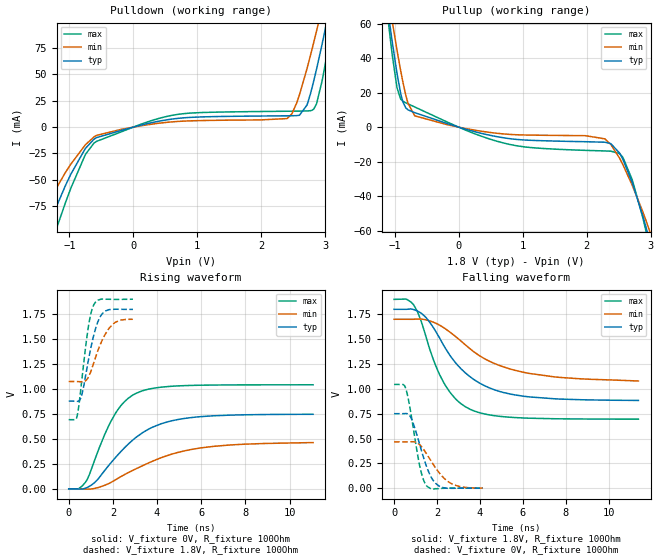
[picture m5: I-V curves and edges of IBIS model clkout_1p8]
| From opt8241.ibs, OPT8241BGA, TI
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|   clkout_1p8 Model
[Model]   clkout_1p8
Model_type   Output
Polarity   Non-Inverting
Vmeas = 0.9
Vref = 0
Cref = 2pF
Rref = 250
|   typ   min   max
|   (nom PVT)   (fast PVT)   (slow PVT)
C_comp   2.233e-12   2.012e-12   2.445e-12
| Where nom  PVT is Nominal Process, 1.8V, 27C
|   Fast PVT is Strong Process,  1.9V, -40C
|   Slow PVT is Weak Process,   1.7V, 125C
[Voltage Range]   1.8   1.7   1.9
|Junction Temperature
[Temperature Range]   27   125   -40
[Pullup Reference]   1.8   1.7   1.9
[Pulldown Reference]   0   0   0
[Power Clamp Reference]   1.8   1.7   1.9
[GND Clamp Reference]   0   0   0
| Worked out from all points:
|   slope of the pulldown table from 0 to 0.27 V, typ, clamps not added: 67 ohm
|   slope of the pullup table from 0 to 0.27 V, typ, clamps not added: 96 ohm
|   falling waveform, V_fixture 1.8V, R_fixture 100Ohm: 20-80 % time 2.09ns typ, 2.79ns min, 1.42ns max; typ from 1.8 V to 0.884 V
|   rising waveform, V_fixture 0V, R_fixture 100Ohm: 20-80 % time 2.11ns typ, 2.92ns min, 1.32ns max; typ from 0 V to 0.747 V
|   rising waveform, V_fixture 1.8V, R_fixture 100Ohm: 20-80 % time 522ps typ, 686ps min, 403ps max; typ from 0.879 V to 1.8 V
|   falling waveform, V_fixture 0V, R_fixture 100Ohm: 20-80 % time 669ps typ, 935ps min, 493ps max; typ from 0.75 V to 0 V
[Pulldown]
|   Voltage   I(typ)   I(min)   I(max)
-1.8V     -252mA     -148.4mA   -354.1mA
-1.551V   -125.9mA   -94.92mA   -164.8mA
-1.06V    -55.32mA   -42.92mA   -71.6mA
-572.4mV  -9.892mA   -7.778mA   -13.42mA
682mV     8.222mA    5.348mA    11.98mA
2.402V    10.74mA    8.113mA    15.09mA
2.596V    11.26mA    30.56mA    15.21mA
2.79V     36.73mA    73.35mA    15.93mA
2.864V    55.26mA    91.37mA    22.36mA
2.968V    83.99mA    117.5mA    49.6mA
3.074V    115.1mA    144.2mA    84.39mA
3.6V      273.5mA    274.3mA    277.1mA
[Pullup]
|   Voltage   I(typ)   I(min)   I(max)
-1.8V     274.1mA    250.5mA    313.5mA
-1.15V    80.37mA    88.29mA    78.6mA
-1.083V   61.49mA    71.92mA    55.92mA
-1.04V    50.09mA    61.9mA     42.54mA
-963.6mV  31.24mA    44.74mA    22.93mA
-872.8mV  14.84mA    26.45mA    15.08mA
-684.8mV  8.358mA    6.543mA    11.66mA
736.4mV   -6.36mA    -4.039mA   -9.499mA
2.285V    -8.738mA   -6.793mA   -13.8mA
2.569V    -18.88mA   -21.91mA   -17.72mA
2.921V    -57.01mA   -53.4mA    -59.13mA
3.6V      -244.1mA   -200.4mA   -264.4mA
[Ramp]
R_load = 100
|   typ   min   max
dV/dt_r   0.448492/2.11362e-09   0.278333/2.92774e-09   0.625405/1.32211e-09
dV/dt_f   0.551164/2.09736e-09   0.372739/2.78836e-09   0.723351/1.41986e-09
[Falling Waveform]
V_fixture = 1.8V
V_fixture_min = 1.7V
V_fixture_max = 1.9V
R_fixture = 100Ohm
|   Time   V(typ)   V(min)   V(max)
0s        1.8V       1.7V       1.9V
552ps     1.8V       1.7V       1.903V
922ps     1.797V     1.7V       1.841V
1.542ns   1.703V     1.691V     1.486V
2.286ns   1.447V     1.619V     1.075V
2.896ns   1.255V     1.521V     893mV
3.536ns   1.123V     1.404V     795.3mV
4.656ns   992.3mV    1.257V     730.8mV
6.22ns    921.1mV    1.158V     705.5mV
11.39ns   883.5mV    1.079V     695.3mV
[Rising Waveform]
V_fixture = 0V
V_fixture_min = 0V
V_fixture_max = 0V
R_fixture = 100Ohm
|   Time   V(typ)   V(min)   V(max)
0s        627pV      37.55nV    314.5pV
432ps     -783.4uV   193.2uV    -141.6uV
762ps     6.722mV    -1.682mV   67.26mV
1.168ns   61.63mV    3.847mV    284.4mV
1.626ns   183.3mV    35.28mV    543.2mV
2.108ns   311.5mV    89.13mV    753.5mV
3.034ns   513mV      199.2mV    954.9mV
4.118ns   646.2mV    305.9mV    1.016V
5.506ns   712.5mV    392.3mV    1.035V
11.07ns   746.6mV    463.3mV    1.042V
[Rising Waveform]
V_fixture = 1.8V
V_fixture_min = 1.7V
V_fixture_max = 1.9V
R_fixture = 100Ohm
|   Time   V(typ)   V(min)   V(max)
0s        878.8mV    1.075V     692.6mV
386ps     875.9mV    1.075V     733.9mV
596ps     944.9mV    1.071V     1.097V
862ps     1.254V     1.108V     1.582V
994ps     1.404V     1.171V     1.745V
1.128ns   1.533V     1.258V     1.84V
1.426ns   1.724V     1.443V     1.897V
1.836ns   1.795V     1.61V      1.898V
2.374ns   1.797V     1.69V      1.897V
2.906ns   1.797V     1.698V     1.898V
[Falling Waveform]
V_fixture = 0V
V_fixture_min = 0V
V_fixture_max = 0V
R_fixture = 100Ohm
|   Time   V(typ)   V(min)   V(max)
0s        750.5mV    466.9mV    1.044V
546ps     751.7mV    466.8mV    1.003V
814ps     697.7mV    468.1mV    716.3mV
1.178ns   452.8mV    442.1mV    242.1mV
1.362ns   318.2mV    395.3mV    91.18mV
1.512ns   219.5mV    347.2mV    25.77mV
1.814ns   81.96mV    244.4mV    -9.017mV
2.17ns    13.76mV    137.9mV    -2.224mV
2.944ns   472.2uV    23.83mV    765.4uV
4.138ns   466.4uV    1.048mV    119.5uV
